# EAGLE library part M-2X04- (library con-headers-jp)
MALE HEADER
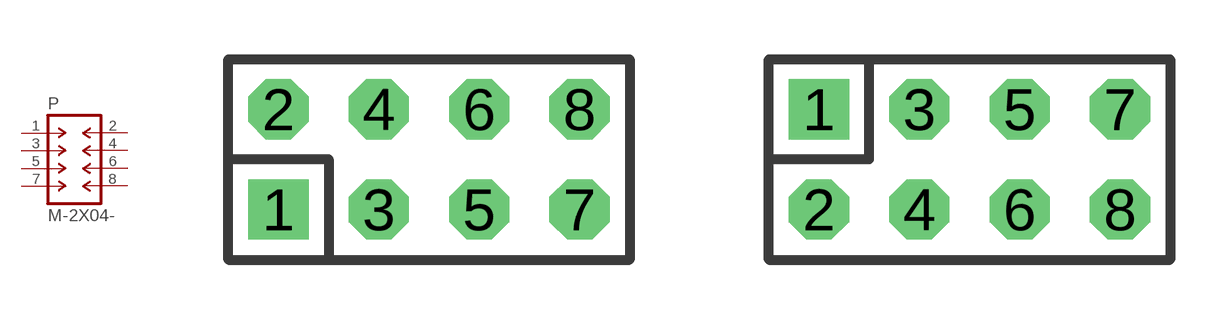
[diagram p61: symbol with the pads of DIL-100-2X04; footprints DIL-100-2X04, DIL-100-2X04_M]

Designator prefix P

## M-2X04-DIL-100  [DIL-100-2X04]
1  1  pas
2  2  pas
3  3  pas
4  4  pas
5  5  pas
6  6  pas
7  7  pas
8  8  pas

## M-2X04-DIL-100_M  [DIL-100-2X04_M]
Pads as for DIL-100-2X04

## M-2X04-DIL-2MM  [DIL-2MM-2X04]
Pads as for DIL-100-2X04

## M-2X04-DIL-2MM_M  [DIL-2MM-2X04_M]
Pads as for DIL-100-2X04

## M-2X04-87759  [87759-08]
Pads as for DIL-100-2X04

## M-2X04-87759_M  [87759-08_M]
Pads as for DIL-100-2X04

## Footprint DIL-100-2X04 (pad centres in mm)
PIN HEADER - 0.1"
drill 1.016 square: 1 -3.81,-1.27
drill 1.016 octagon: 2 -3.81,1.27; 3 -1.27,-1.27; 4 -1.27,1.27; 5 1.27,-1.27; 6 1.27,1.27; 7 3.81,-1.27; 8 3.81,1.27

## Footprint DIL-100-2X04_M (pad centres in mm)
PIN HEADER - MIRRORED 0.1"
drill 1.016 square: 1 -3.81,1.27
drill 1.016 octagon: 2 -3.81,-1.27; 3 -1.27,1.27; 4 -1.27,-1.27; 5 1.27,1.27; 6 1.27,-1.27; 7 3.81,1.27; 8 3.81,-1.27

## Footprint DIL-2MM-2X04 (pad centres in mm)
PIN HEADER - 2MM"
drill 0.711 square: 1 -3,-1
drill 0.711: 2 -3,1; 3 -1,-1; 4 -1,1; 5 1,-1; 6 1,1; 7 3,-1; 8 3,1

## Footprint DIL-2MM-2X04_M (pad centres in mm)
PIN HEADER - MIRRORED 2MM
drill 0.711 square: 1 -3,1
drill 0.711: 2 -3,-1; 3 -1,1; 4 -1,-1; 5 1,1; 6 1,-1; 7 3,1; 8 3,-1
